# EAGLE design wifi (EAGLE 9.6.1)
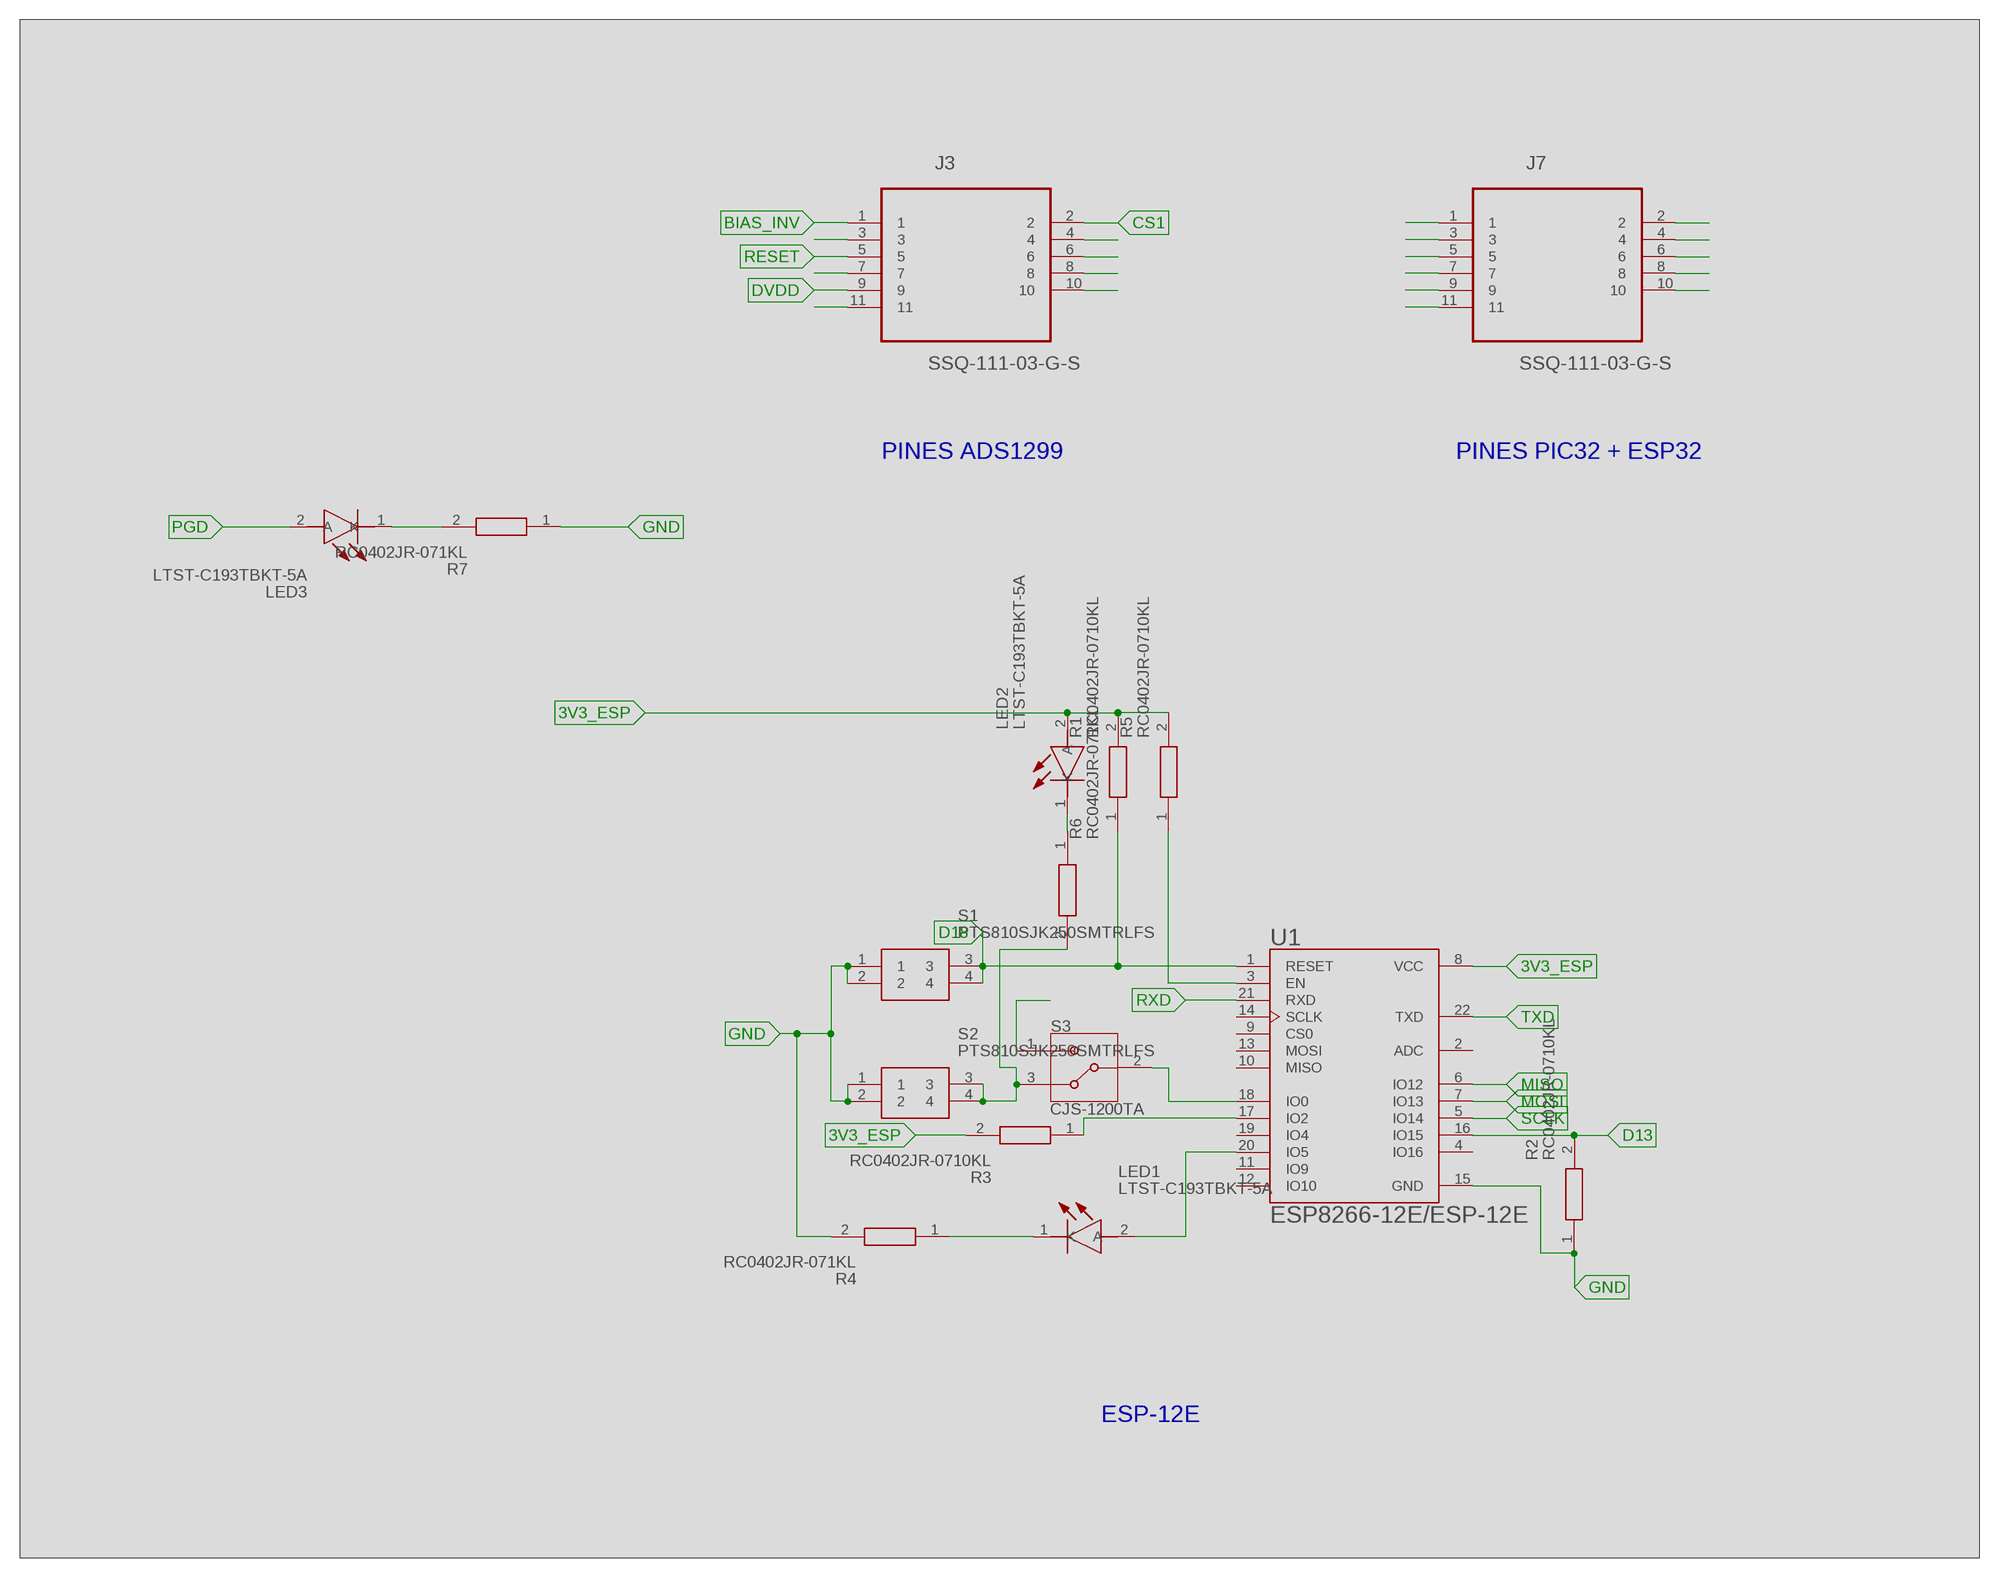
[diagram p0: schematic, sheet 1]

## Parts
J3  SSQ-111-03-G-S  [SAMTEC_SSQ-111-03-G-S]
J7  SSQ-111-03-G-S  [SAMTEC_SSQ-111-03-G-S]
LED1  LTST-C193TBKT-5A  [LEDC1608X45N]
LED2  LTST-C193TBKT-5A  [LEDC1608X45N]
LED3  LTST-C193TBKT-5A  [LEDC1608X45N]
R1  RC0402JR-0710KL  [RESC1005X40N]
R2  RC0402JR-0710KL  [RESC1005X40N]
R3  RC0402JR-0710KL  [RESC1005X40N]
R4  RC0402JR-071KL  [RESC1005X40N]
R5  RC0402JR-0710KL  [RESC1005X40N]
R6  RC0402JR-071KL  [RESC1005X40N]
R7  RC0402JR-071KL  [RESC1005X40N]
S1  PTS810SJK250SMTRLFS  [PTS810SJG250SMTRLFS]
S2  PTS810SJK250SMTRLFS  [PTS810SJG250SMTRLFS]
S3  CJS-1200TA  [SW_CJS-1200TA]
U1  ESP8266-12E/ESP-12E  [XCVR_ESP8266-12E/ESP-12E]

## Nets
3V3_ESP: J7.2 LED2.2(A) R1.2 R3.2 R5.2 U1.8(VCC)
AVDD: J3.10
AVSS: J3.11
BIAS_INV: J3.1
BOOT_EN: J3.6
CLK: J3.4
CS1: J3.2
CS2: J3.3
D13: J3.7 R2.2 U1.16(IO15)
D18: J3.8 R1.1 S1.3 S1.4 U1.1(RESET)
DVDD: J3.9
GND: J7.3 R2.1 R4.2 R7.1 S1.1 S1.2 S2.1 S2.2 U1.15(GND)
GPIO0: J7.11 S3.1
MCLR: J7.1
MISO: J7.7 U1.6(IO12)
MOSI: J7.8 U1.7(IO13)
N$1: S3.2 U1.18(IO0)
N$2: LED1.1(K) R4.1
N$3: R5.1 U1.3(EN)
N$4: LED3.1(K) R7.2
N$5: R6.2 S2.3 S2.4 S3.3
N$6: LED2.1(K) R6.1
N$14: R3.1 U1.17(IO2)
N$15: LED1.2(A) U1.20(IO5)
PGC: J7.5
PGD: J7.4 LED3.2(A)
RESET: J3.5
RXD: J7.9 U1.21(RXD)
SCLK: J7.6 U1.5(IO14)
TXD: J7.10 U1.22(TXD)
Unconnected: U1.2(ADC) U1.4(IO16) U1.9(CS0) U1.10(MISO) U1.11(IO9) U1.12(IO10) U1.13(MOSI) U1.14(SCLK) U1.19(IO4)

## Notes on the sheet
- PINES ADS1299 | PINES PIC32 + ESP32
- ESP-12E

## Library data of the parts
J3 J7 = Cyton:SSQ-111-03-G-S: CONN SOCKET, 2.54MM, THT VERT, 11POS; AVAILABILITY: Unavailable; DESCRIPTION: SSQ Series .100 Tiger Buy™ Socket Strip, Square Tail; MF: Samtec; MP: SSQ-111-03-G-S; PACKAGE: None; PRICE: None
LED1-LED3 = Cyton:LTST-C193TBKT-5A: Standard LEDs - SMD Blue 470nm 28mcd 20mA; DESCRIPTION: Standard LEDs - SMD Blue 470nm 28mcd 20mA; HEIGHT: 0.45mm; MANUFACTURER_NAME: Lite-On; MANUFACTURER_PART_NUMBER: LTST-C193TBKT-5A; RS_PART_NUMBER: 6921051; RS_PRICE-STOCK: https://uk.rs-online.com/web/p/products/6921051
R1-R3 R5 = Cyton:RC0402JR-0710KL: YAGEO (PHYCOMP) - RC0402JR-0710KL - RES, THICK FILM, 10K, 5%, 0.0625W, 0402; DESCRIPTION: YAGEO (PHYCOMP) - RC0402JR-0710KL - RES, THICK FILM, 10K, 5%, 0.0625W, 0402; HEIGHT: 0.4mm; MANUFACTURER_NAME: YAGEO (PHYCOMP); MANUFACTURER_PART_NUMBER: RC0402JR-0710KL
R4 R6 R7 = Cyton:RC0402JR-071KL: YAGEO (PHYCOMP) - RC0402JR-071KL - RES, THICK FILM, 1K, 5%, 0.0625W, 0402; DESCRIPTION: YAGEO (PHYCOMP) - RC0402JR-071KL - RES, THICK FILM, 1K, 5%, 0.0625W, 0402; HEIGHT: 0.4mm; MANUFACTURER_NAME: YAGEO (PHYCOMP); MANUFACTURER_PART_NUMBER: RC0402JR-071KL
S1 S2 = Cyton:PTS810SJK250SMTRLFS: IP40 Black Button Tactile Switch, SPST-NO 50 mA 3mm Surface Mount Source: Datasheet; DESCRIPTION: IP40 Black Button Tactile Switch, SPST-NO 50 mA 3mm Surface Mount; HEIGHT: mm; MANUFACTURER_NAME: C & K COMPONENTS; MANUFACTURER_PART_NUMBER: PTS810SJK250SMTRLFS; RS_PART_NUMBER: 1359396P; RS_PRICE-STOCK: http://uk.rs-online.com/web/p/products/1359396P
S3 = Cyton:CJS-1200TA: Switch Slide N.O./N.C. SPDT Raised Slide 0.1A 24VDC J-Hook SMD Embossed T/R; AVAILABILITY: Unavailable; DESCRIPTION: Slide Switch SPDT Surface Mount; MF: Nidec Copal; MP: CJS-1200TA; PACKAGE: None; PRICE: None
U1 = Cyton:ESP8266-12E/ESP-12E: ESP-12E WiFi Module; AVAILABILITY: Unavailable; DESCRIPTION: This WiFi module has a 32-bit MCU micro and clock speeds supporting 80 MHz or 160 MHz. Supports the RTOS and integrated Wi-Fi MAC/BB/RF/PA/LNA, and has an on-board antenna.; MF: AI-Thinker; MP: ESP8266-12E/ESP-12E; PACKAGE: None; PRICE: None

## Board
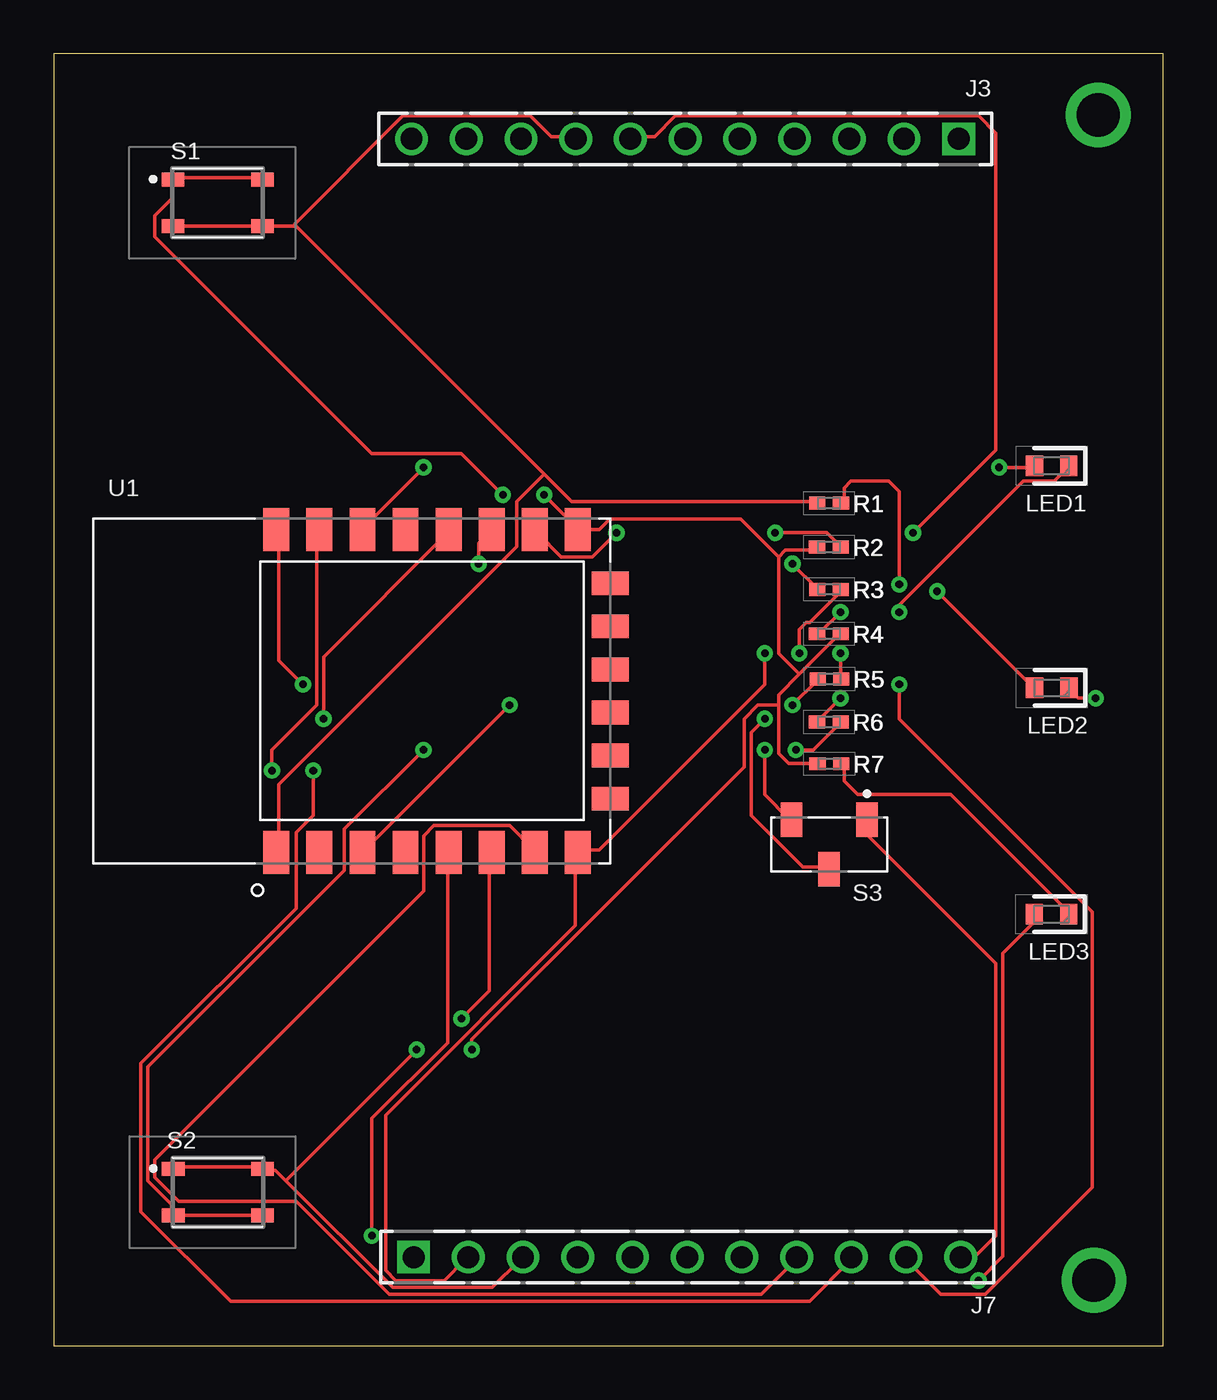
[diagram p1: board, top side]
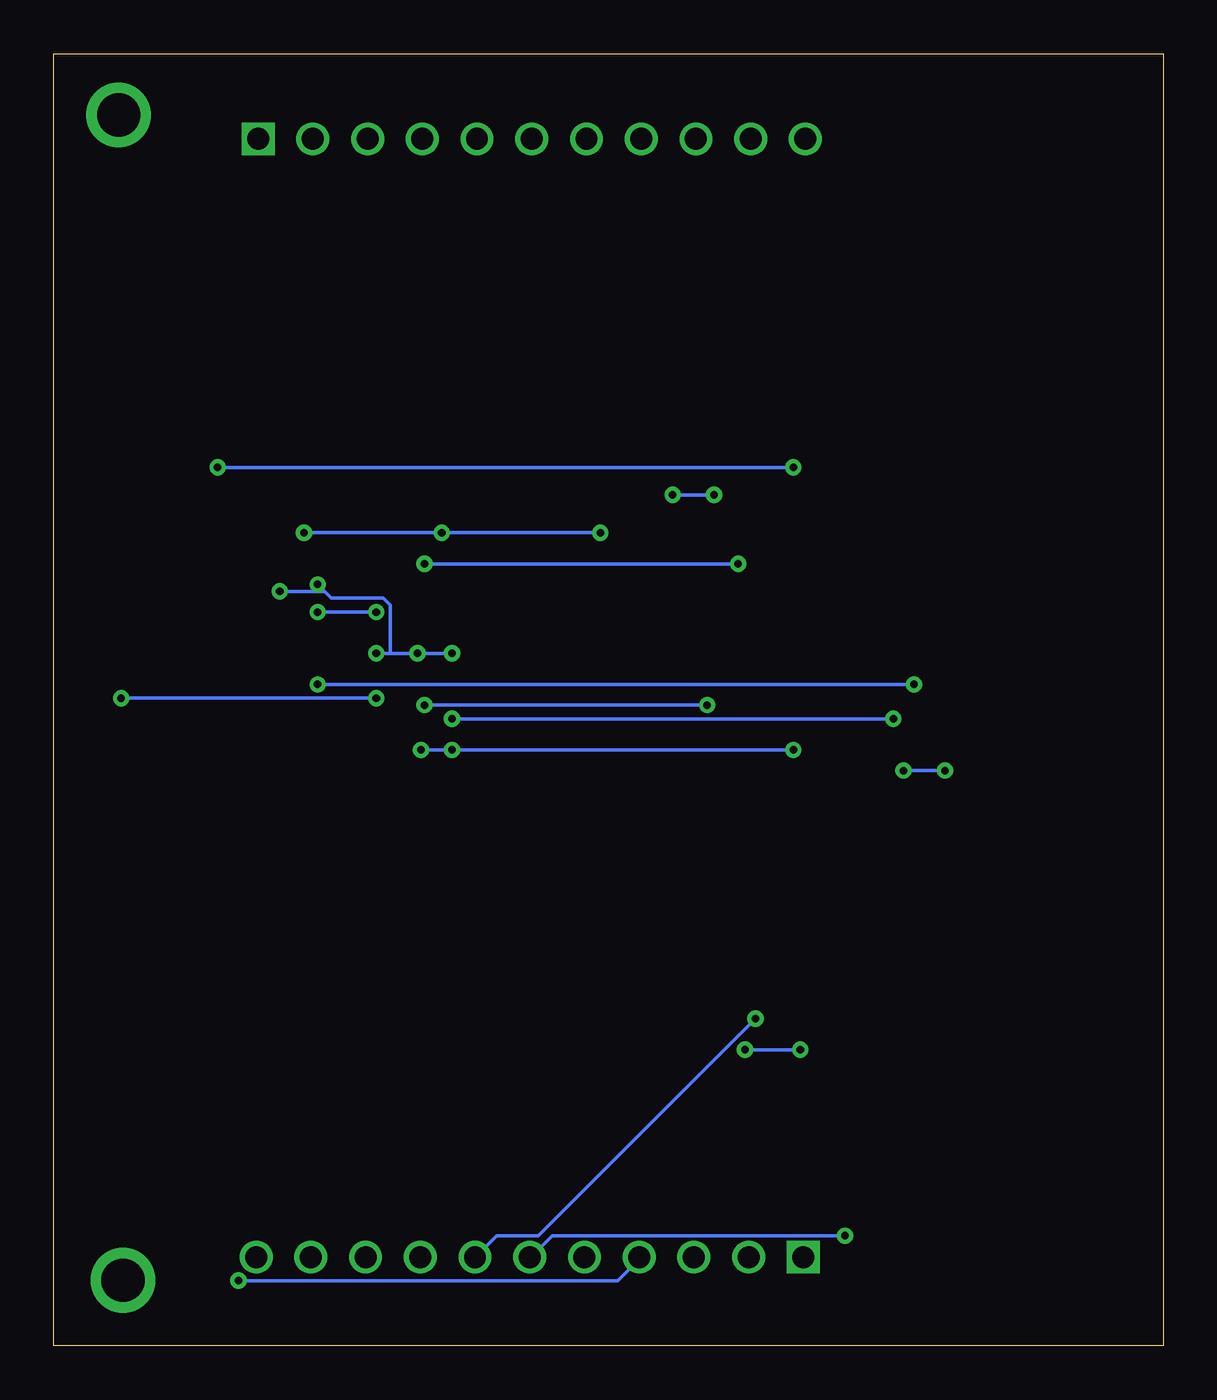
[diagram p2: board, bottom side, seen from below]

Size 51.48 x 59.98 mm. Coordinates in mm from the lower left corner, seen from the top.
Outline: 0,0 51.48,0 51.48,59.98 0,59.98 0,0
Copper layers (1*16): Top 0.035mm / dielectric 1.5mm / Bottom 0.035mm
Design rules "default *": minimum track width 6mil, minimum drill 0.35mm, track to track 6mil, track to pad 6mil, pad to pad 6mil, via to via 6mil, smd to smd 6mil, copper to edge 40mil, drill to drill 6mil, minimum pad ring 10mil, minimum via ring 8mil, stop-mask expansion 0mil, vias tented up to drill 100mil, thermal gap 10mil

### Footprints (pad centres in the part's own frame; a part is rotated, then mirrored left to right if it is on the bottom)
SAMTEC_SSQ-111-03-G-S = drill 1.016 square: 1 -25.4,0 | drill 1.016: 2 -22.86,0; 3 -20.32,0; 4 -17.78,0; 5 -15.24,0; 6 -12.7,0; 7 -10.16,0; 8 -7.62,0; 9 -5.08,0; 10 -2.54,0; 11 0,0
LEDC1608X45N = smd 0.8 x 0.95: 1 -0.8,0; 2 0.8,0
RESC1005X40N = smd 0.75 x 0.6: 1 -0.55,0; 2 0.55,0
PTS810SJG250SMTRLFS = smd 1.05 x 0.65: 1 -2.075,1.075; 2 2.075,1.075; 3 -2.075,-1.075; 4 2.075,-1.075
SW_CJS-1200TA = smd 1 x 1.6: 1 -1.75,-1.15; 2 0,1.15; 3 1.75,-1.15
XCVR_ESP8266-12E/ESP-12E = smd 2 x 1.2: 1 -7.5,7; 2 -7.5,5; 3 -7.5,3; 4 -7.5,1; 5 -7.5,-1; 6 -7.5,-3; 7 -7.5,-5; 8 -7.5,-7; 15 7.5,-7; 16 7.5,-5; 17 7.5,-3; 18 7.5,-1; 19 7.5,1; 20 7.5,3; 21 7.5,5; 22 7.5,7 | smd 1.1 x 1.7: 9 -5,-8.5; 10 -3,-8.5; 11 -1,-8.5; 12 1,-8.5; 13 3,-8.5; 14 5,-8.5

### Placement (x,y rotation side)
J3  16.6,56.04 180 top
J7  42.1,4.11 0 top
LED1  46.31,40.85 180 top
LED2  46.32,30.54 180 top
LED3  46.31,20.04 180 top
R1  35.99,39.12 0 top
R2  35.97,37.08 0 top
R3  35.98,35.12 0 top
R4  35.97,33.05 0 top
R5  36,30.96 0 top
R6  35.97,28.96 0 top
R7  35.99,27.02 0 top
S1  7.6,53.06 0 top
S2  7.62,7.13 0 top
S3  35.99,23.27 180 top
U1  17.33,30.4 90 top

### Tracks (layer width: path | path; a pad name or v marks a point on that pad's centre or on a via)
3V3_ESP  (via drill 0.35)
  Top 0.152: v34.6,32.14 34.6,33.26 34.92,33.58 35.08,33.58 36.52,35.02 R3.2 | v36.52,32.14 36.52,31.02 R5.2 | v39.24,35.34 39.24,39.66 38.76,40.14 37,40.14 36.68,39.82 36.68,39.18 R1.2 | v41,35.02 45.48,30.54 LED2.2 | J7.2 19.08,3.98 18.12,3.02 15.88,3.02 15.4,3.5 15.4,10.7 24.2,19.5 24.2,22.86 U1.8 24.36,23.02 25.32,23.02 33,30.7 v33,32.14
  Bottom 0.152: v36.52,32.14 35.88,32.14 | 35.88,32.14 v34.6,32.14 v33,32.14 | 38.92,35.02 38.6,34.7 36.2,34.7 35.88,34.38 35.88,32.14 | 38.92,35.02 v39.24,35.34 | 38.92,35.02 v41,35.02
D13  (via drill 0.35)
  Top 0.152: v33.48,37.74 35.88,37.74 36.52,37.1 R2.2 | v26.12,37.74 25,36.62 23.56,36.62 22.44,37.74 U1.16 | v39.88,37.74 43.72,41.58 43.72,56.3 42.92,57.1 28.84,57.1 27.88,56.14 26.92,56.14 J3.7
  Bottom 0.152: v26.12,37.74 v33.48,37.74 v39.88,37.74
D18
  Top 0.152: 22.76,40.46 11.24,51.98 11.08,51.98 | 22.76,40.46 24.04,39.18 35.4,39.18 R1.1 | 11.08,51.98 9.8,51.98 S1.4 9.64,51.98 5.64,51.98 S1.3 | 22.76,40.46 21.48,39.18 21.48,37.1 10.44,26.06 10.44,23.02 U1.1 | 11.08,51.98 16.2,57.1 22.12,57.1 23.08,56.14 24.2,56.14 J3.8
GND  (via drill 0.35)
  Top 0.152: S2.1 5.64,8.3 9.64,8.3 S2.2 9.8,8.14 10.28,8.14 10.76,7.66 | 10.76,7.66 15.72,2.7 20.36,2.7 21.64,3.98 J7.3 | S1.2 9.64,54.22 5.64,54.22 S1.1 5.48,54.06 5.48,53.26 4.68,52.46 4.68,51.5 14.76,41.42 18.92,41.42 v20.84,39.5 | 33.64,29.74 33.64,30.22 34.6,31.18 | 33.64,29.74 33.64,27.5 34.12,27.02 35.4,27.02 R7.1 | 34.6,31.18 36.52,33.1 R4.2 | 33.64,36.62 33.96,36.94 35.4,36.94 R2.1 | 33.64,36.62 33.64,32.14 34.6,31.18 | 24.36,37.9 25.32,37.9 25.8,38.38 31.88,38.38 33.64,36.62 | 24.36,37.9 v22.76,39.5 | 24.36,37.9 U1.15 | v16.84,13.74 10.76,7.66 | v19.4,13.74 19.4,14.22 32.04,26.86 32.04,29.1 32.68,29.74 33.64,29.74
  Bottom 0.152: v22.76,39.5 v20.84,39.5 | v19.4,13.74 v16.84,13.74
GPIO0
  Top 0.152: S3.1 37.8,24.3 37.8,23.66 43.72,17.74 43.72,5.1 42.76,4.14 42.12,4.14 J7.11
MISO  (via drill 0.35)
  Top 0.152: v18.92,15.18 20.2,16.46 20.2,22.86 U1.6
  Bottom 0.152: v18.92,15.18 29,5.1 30.92,5.1 31.88,4.14 J7.7
MOSI
  Top 0.152: U1.7 22.28,23.02 21.16,24.14 17.64,24.14 17.16,23.66 17.16,21.1 4.68,8.62 4.68,7.82 5.8,6.7 11.24,6.7 15.56,2.38 32.84,2.38 34.44,3.98 J7.8
N$1  (via drill 0.35)
  Top 0.152: v33,29.1 32.36,28.46 32.36,24.62 34.76,22.22 35.88,22.22 S3.2 | v12.52,29.1 12.52,31.98 18.28,37.74 U1.18
  Bottom 0.152: v12.52,29.1 v33,29.1
N$2  (via drill 0.35)
  Top 0.152: v36.52,34.06 35.56,33.1 R4.1 | v39.24,34.06 39.24,34.38 45,40.14 46.44,40.14 47.08,40.78 LED1.1
  Bottom 0.152: v39.24,34.06 v36.52,34.06
N$3  (via drill 0.35)
  Top 0.152: v34.28,29.74 35.4,30.86 R5.1 | v21.16,29.74 14.44,23.02 U1.3
  Bottom 0.152: v21.16,29.74 v34.28,29.74
N$4
  Top 0.152: R7.2 36.68,26.86 36.68,26.22 37.32,25.58 41.64,25.58 47.08,20.14 LED3.1
N$5  (via drill 0.35)
  Top 0.152: S2.4 9.64,6.06 5.64,6.06 S2.3 5.48,6.06 5.48,6.54 4.36,7.66 4.36,12.94 13.48,22.06 13.48,23.98 v17.16,27.66 | v34.44,27.66 35.24,27.66 36.52,28.94 R6.2 | v33,27.66 33,25.58 34.12,24.46 S3.3
  Bottom 0.152: v34.44,27.66 v33,27.66 v17.16,27.66
N$6  (via drill 0.35)
  Top 0.152: v36.52,30.06 35.56,29.1 R6.1 | v48.36,30.06 47.56,30.06 47.24,30.38 LED2.1
  Bottom 0.152: v48.36,30.06 v36.52,30.06
N$8  (via drill 2 pad 3)
  other vias: 48.27,3.04
N$9  (via drill 2 pad 3)
  other vias: 48.48,57.15
N$14  (via drill 0.35)
  Top 0.152: v34.28,36.3 35.4,35.18 R3.1 | v19.72,36.3 19.72,37.26 20.2,37.74 U1.17
  Bottom 0.152: v19.72,36.3 v34.28,36.3
N$15  (via drill 0.35)
  Top 0.152: v43.88,40.78 45.48,40.78 LED1.2 | v17.16,40.78 14.28,37.9 U1.20
  Bottom 0.152: v17.16,40.78 v43.88,40.78
PGD  (via drill 0.35)
  Top 0.152: v42.92,3.02 44.04,4.14 44.04,18.22 45.48,19.66 45.48,19.98 LED3.2
  Bottom 0.152: v42.92,3.02 25.32,3.02 24.36,3.98 J7.4
RXD  (via drill 0.35)
  Top 0.152: v10.12,26.7 10.12,27.66 12.2,29.74 12.2,37.74 U1.21 | v12.04,26.7 12.04,24.62 11.24,23.82 11.24,20.3 4.04,13.1 4.04,6.22 8.2,2.06 35.08,2.06 37,3.98 J7.9
  Bottom 0.152: v12.04,26.7 v10.12,26.7
SCLK  (via drill 0.35)
  Top 0.152: v14.76,5.1 14.76,10.54 18.28,14.06 18.28,22.86 U1.5
  Bottom 0.152: v14.76,5.1 28.36,5.1 29.32,4.14 J7.6
TXD  (via drill 0.35)
  Top 0.152: v11.56,30.7 10.44,31.82 10.44,37.74 U1.22 | v39.24,30.7 39.24,29.1 48.2,20.14 48.2,7.34 43.24,2.38 41.16,2.38 39.56,3.98 J7.10
  Bottom 0.152: v39.24,30.7 v11.56,30.7

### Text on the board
space: AVSS | AVDD | DVDD | WIFI-RST | ESP-SS | EN | ADS-RST | CLK | CS2 | CS1 | BIAS-INV | MCLR | 3V3 | GND | PGD | PGC | SCLK | MISO | MOSI | RXD | TXD | GPIO0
